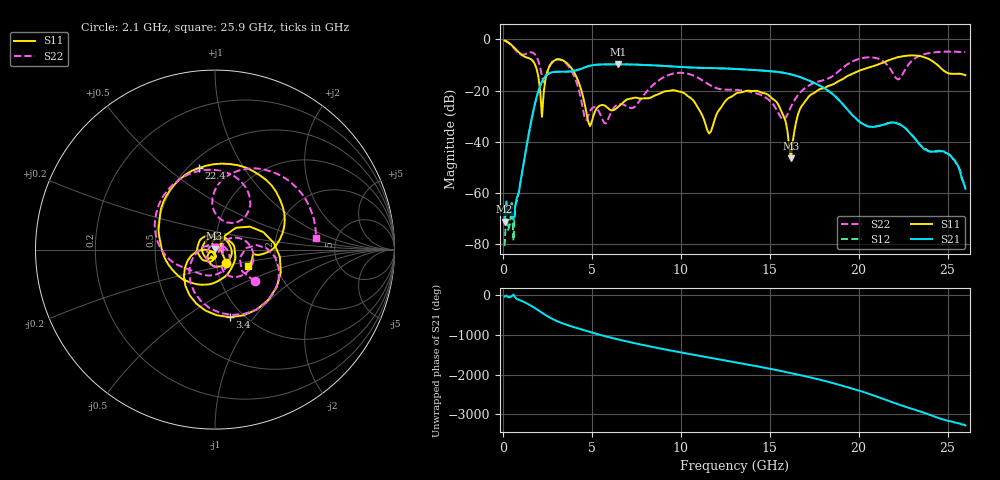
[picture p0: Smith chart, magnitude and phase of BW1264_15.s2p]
!Keysight Technologies,N5245B,MY57181159,A.13.60.06
!Date: Friday, December 18, 2020 23:52:41
!Correction: S11(Full 2 Port(1,2))
!S21(Full 2 Port(1,2))
!S12(Full 2 Port(1,2))
!S22(Full 2 Port(1,2))
!S2P File: Measurements: S11, S21, S12, S22:
# Hz S  dB  R 50
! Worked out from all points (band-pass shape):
!   260 points, 100 MHz to 26 GHz, reference 50 ohm
!   highest |S21| = -9.73 dB at 6.5 GHz (marker M1); lowest = -71.3 dB at 100 MHz (marker M2)
!   |S21| within 3 dB of the highest: 2.863 GHz to 15.48 GHz (12.62 GHz wide, 138 % of centre)
!   lowest |S11| = -46.5 dB at 16.2 GHz (marker M3), VSWR 1.01, Z = 49.8 + j0.428 ohm
!   |S11| at or under -10 dB: 1.819 GHz to 2.669 GHz (850.6 MHz wide, 37.9 % of centre); 3.707 GHz to 21.02 GHz (17.31 GHz wide, 140 % of centre); 24.43 GHz to end of sweep
!   |S22| runs from -32.8 to -0.4 dB; largest |S21 - S12| = 0.00057
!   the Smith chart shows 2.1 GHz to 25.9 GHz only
!   S11 on the Smith chart (normalised r, x): 2.1 GHz: 1.12, -0.17; 3.4 GHz: 0.87, -0.77; 22.4 GHz: 0.56, +0.65; 25.9 GHz: 1.42, -0.27
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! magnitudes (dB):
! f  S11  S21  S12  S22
! 100 MHz  -0.4  -71.3  -80.9  -0.4
! 500 MHz  -2.3  -67.6  -63.2  -2.5
! 600 MHz  -2.9  -70.6  -78.7  -3.3
! 700 MHz  -3.6  -65.2  -64.9  -4.1
! 2.1 GHz  -20.3  -18.1  -18.1  -10.9
! 2.2 GHz  -30.3  -16.5  -16.5  -14.3
! 2.5 GHz  -12.7  -13.7  -13.7  -12.6
! 3.4 GHz  -8.3  -12.7  -12.7  -8.5
! 4.5 GHz  -22.2  -11.2  -11.2  -27.2
! 4.9 GHz  -33.9  -10.3  -10.3  -28.1
! 6.5 GHz  -26.3  -9.7  -9.7  -25.4
! 8.8 GHz  -21.3  -10.3  -10.2  -15.8
! 11.6 GHz  -36.8  -11.2  -11.2  -17.7
! 13.1 GHz  -21.2  -11.5  -11.5  -19.7
! 15.4 GHz  -24.6  -12.7  -12.6  -27.7
! 16.2 GHz  -46.5  -13.7  -13.7  -26.2
! 16.6 GHz  -29.2  -14.5  -14.5  -21.6
! 17.4 GHz  -21.3  -16.7  -16.7  -17.3
! 21.7 GHz  -8.1  -32.7  -32.7  -10.8
! 22.4 GHz  -6.7  -33.6  -33.5  -14.4
! 25.9 GHz  -13.7  -56.1  -55.9  -4.9
! 26 GHz  -14.0  -58.4  -58.1  -5.0
